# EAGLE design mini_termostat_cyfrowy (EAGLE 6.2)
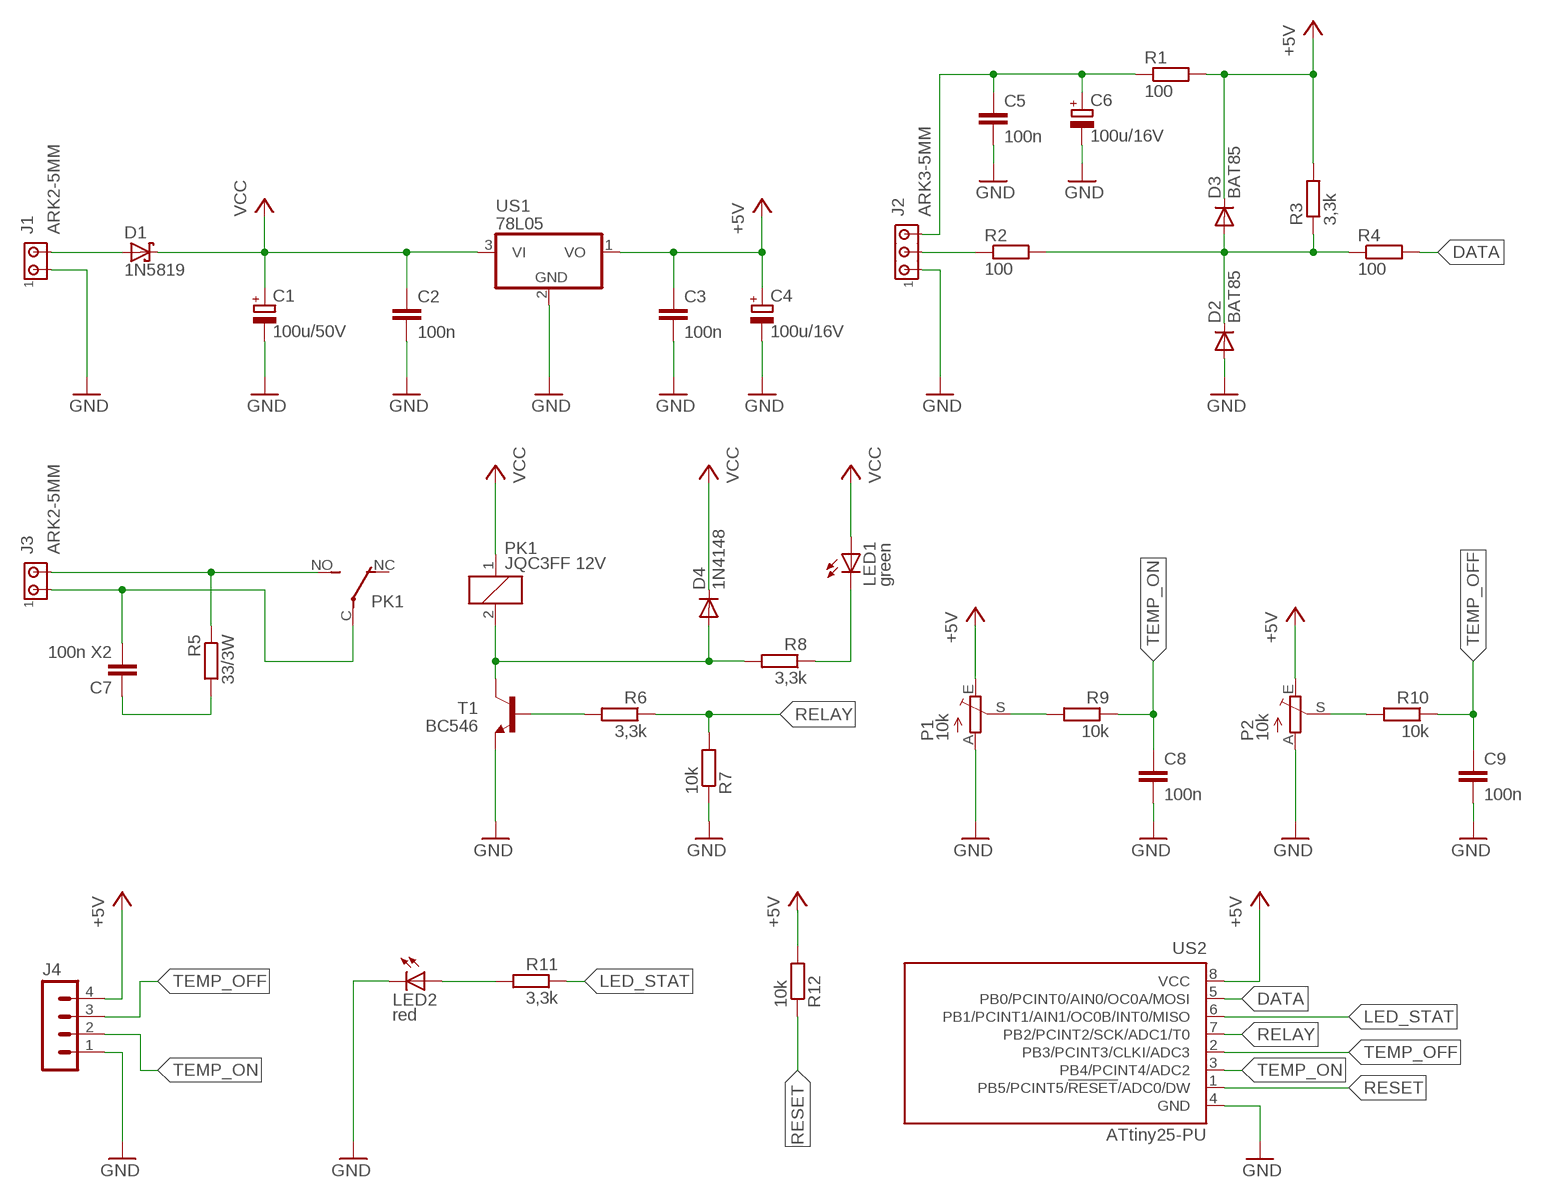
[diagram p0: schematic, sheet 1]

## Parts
C1  100u/50V  CPOL-EUE3.5-8  [E3,5-8]
C2  100n  C-EU050-025X075  [C050-025X075]
C3  100n  C-EU050-025X075  [C050-025X075]
C4  100u/16V  CPOL-EUE2.5-6  [E2,5-6]
C5  100n  C-EU050-025X075  [C050-025X075]
C6  100u/16V  CPOL-EUE2.5-5  [E2,5-5]
C7  100n X2  C-EU102_152-062X184  [C102_152-062X184]
C8  100n  C-EU050-025X075  [C050-025X075]
C9  100n  C-EU050-025X075  [C050-025X075]
D1  1N5819  1N5819-T  [DO41-7.6]
D2  BAT85  BAT81  [DO34-7]
D3  BAT85  BAT81  [DO34-7]
D4  1N4148  BAT81  [DO34-7]
J1  ARK2-5MM  [2PIN-5MM]
J2  ARK3-5MM  [3PIN-5MM]
J3  ARK2-5MM  [2PIN-5MM]
J4  MA04-1  [MA04-1]
LED1  green  LED5MM  [LED5MM]
LED2  red  LED5MM  [LED5MM]
P1  10k  TRIM_EU-B64Y  [B64Y]
P2  10k  TRIM_EU-B64Y  [B64Y]
PK1  JQC3FF 12V  PK_POJED-JQC-3FG  [PK_POJED_JQC-3FG]
R1  100  R-EU_0207/7  [0207/7]
R2  100  R-EU_0207/7  [0207/7]
R3  3,3k  R-EU_0204/2V  [0204V]
R4  100  R-EU_0207/7  [0207/7]
R5  33/3W  R-EU_0617/5V  [0617V]
R6  3,3k  R-EU_0207/7  [0207/7]
R7  10k  R-EU_0207/7  [0207/7]
R8  3,3k  R-EU_0204/2V  [0204V]
R9  10k  R-EU_0207/7  [0207/7]
R10  10k  R-EU_0207/7  [0207/7]
R11  3,3k  R-EU_0204/2V  [0204V]
R12  10k  R-EU_0204/2V  [0204V]
T1  BC546  BC546A  [TO92-EBC]
US1  78L05  7805L  [TO92]
US2  ATtiny25-PU  TINY13-20PU  [DIL08]

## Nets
+5V: C3.1 C4.+ D3.C J4.4 P1.E P2.E R1.2 R3.2 R12.2 US1.1(VO) US2.8(VCC)
DATA: R4.2 US2.5(PB0/PCINT0/AIN0/OC0A/MOSI)
GND: C1.- C2.2 C3.2 C4.- C5.2 C6.- C8.2 C9.2 D2.A J1.P$1 J2.P$1 J4.1 LED2.K(C) P1.A P2.A R7.1 T1.E US1.2(GND) US2.4(GND)
LED_STAT: R11.1 US2.6(PB1/PCINT1/AIN1/OC0B/INT0/MISO)
N$1: D1.A J1.P$2
N$2: J3.P$2 PK1.NO R5.1
N$3: P1.S R9.2
N$4: P2.S R10.2
N$5: LED1.K(C) R8.1
N$6: LED2.A R11.2
N$7: R6.2 T1.B
N$9: D4.A PK1.2 R8.2 T1.C
N$11: C7.2 J3.P$1 PK1.C(COM)
N$12: C7.1 R5.2
N$28: C5.1 C6.+ J2.P$3 R1.1
N$29: D2.C D3.A R2.2 R3.1 R4.1
N$30: J2.P$2 R2.1
RELAY: R6.1 R7.2 US2.7(PB2/PCINT2/SCK/ADC1/T0)
RESET: R12.1 US2.1(PB5/PCINT5/!RESET!/ADC0/DW)
TEMP_OFF: C9.1 J4.3 R10.1 US2.2(PB3/PCINT3/CLKI/ADC3)
TEMP_ON: C8.1 J4.2 R9.1 US2.3(PB4/PCINT4/ADC2)
VCC: C1.+ C2.1 D1.C D4.C LED1.A PK1.1 US1.3(VI)
Unconnected: PK1.NC

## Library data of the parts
C1 C4 C6 = rcl:CPOL-EU: POLARIZED CAPACITOR, European symbol
C2 C3 C5 C7-C9 = rcl:C-EU: CAPACITOR, European symbol
D1 = diode:1N581*: 1.0A SCHOTTKY BARRIER RECTIFIER
D2-D4 = diode:BAT81: DIODE
J1 J3 = zlacza_futrzak:ARK2: ARK 2
J2 = zlacza_futrzak:ARK3: ARK 3 Raster 5mm i 3,5mm
J4 = zlacza_futrzak:MA04-1: PIN HEADER; OC_FARNELL: unknown; OC_NEWARK: unknown
LED1 LED2 = led:LED: LED
P1 P2 = pot:TRIM_EU-: POTENTIOMETER
PK1 = inne_futrzak:PK_POJED
R1-R12 = rcl:R-EU_: RESISTOR, European symbol
T1 = transistor-npn:BC546*: NPN Transistor
US1 = linear:78*: Positive VOLTAGE REGULATOR Source: http://cache.national.com/ds/LM/LM78L05.pdf http://www.fairchildsemi.com/ds/LM/LM7805.pdf
US2 = atmel:TINY13: 8-bit AVR Microcontroller with 1K Bytes In-System Programmable Flash Source: http://www.atmel.com/dyn/resources/prod_documents/2535S.pdf; MPN: ATTINY13-20PU; OC_FARNELL: 9171550; OC_NEWARK: 96K6521

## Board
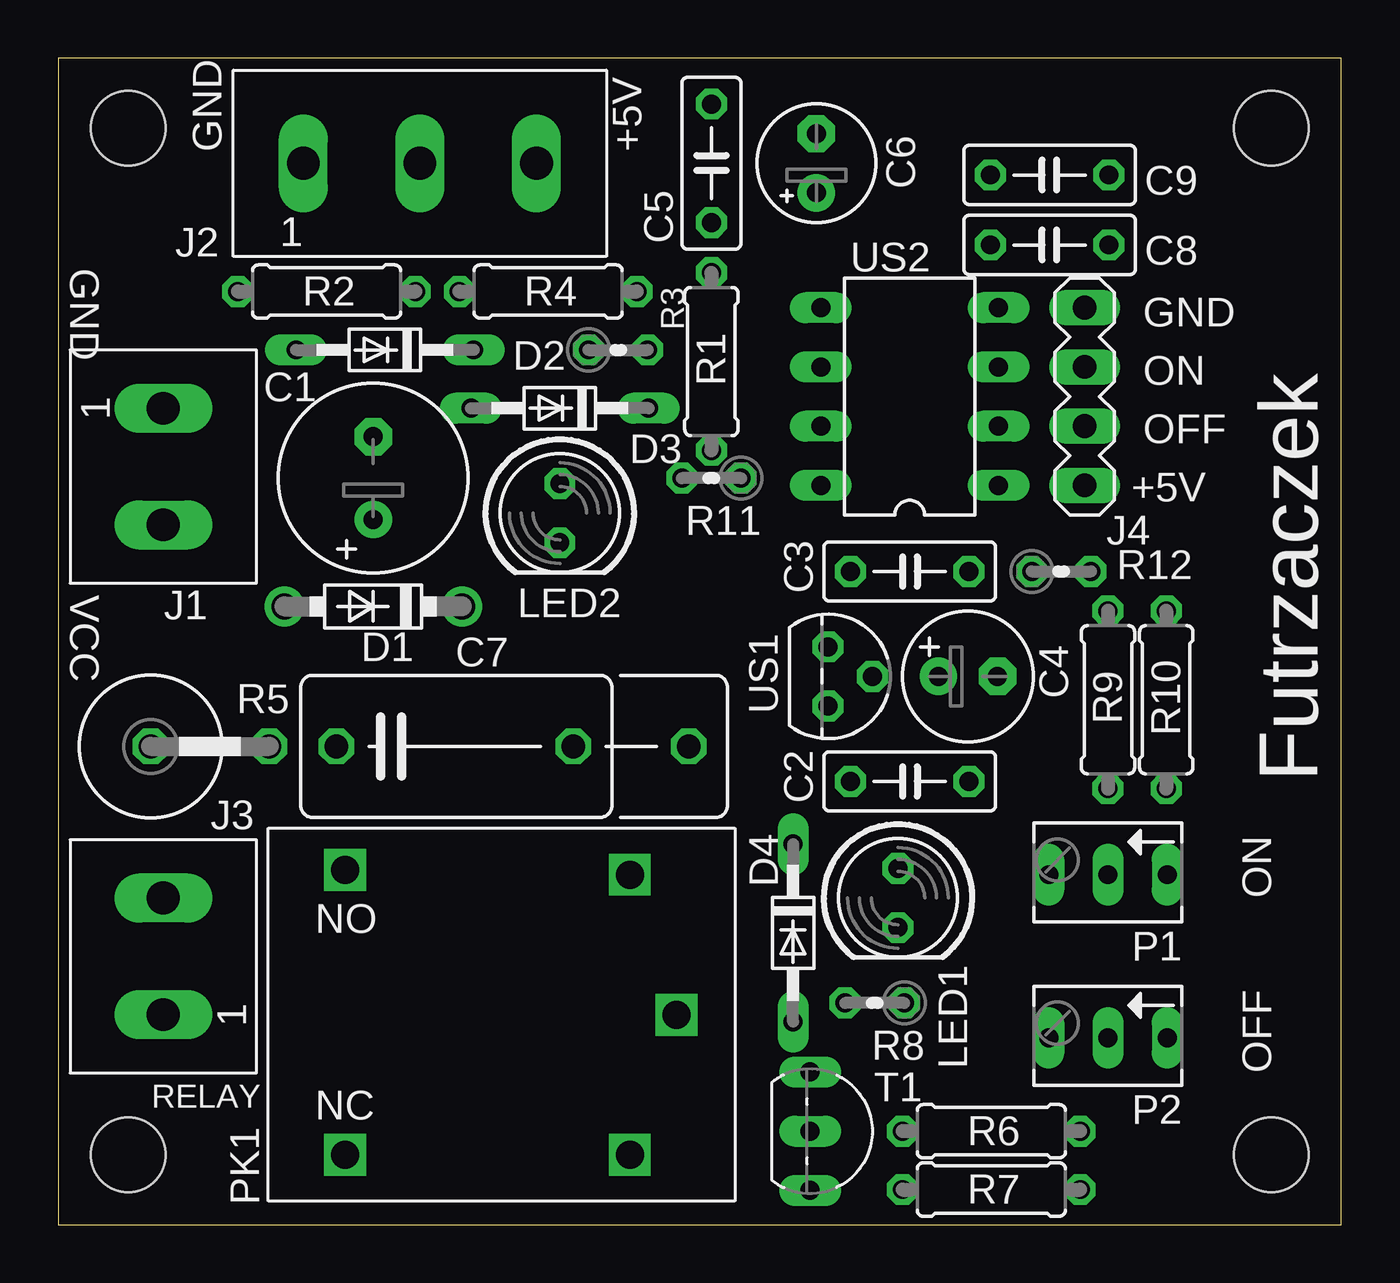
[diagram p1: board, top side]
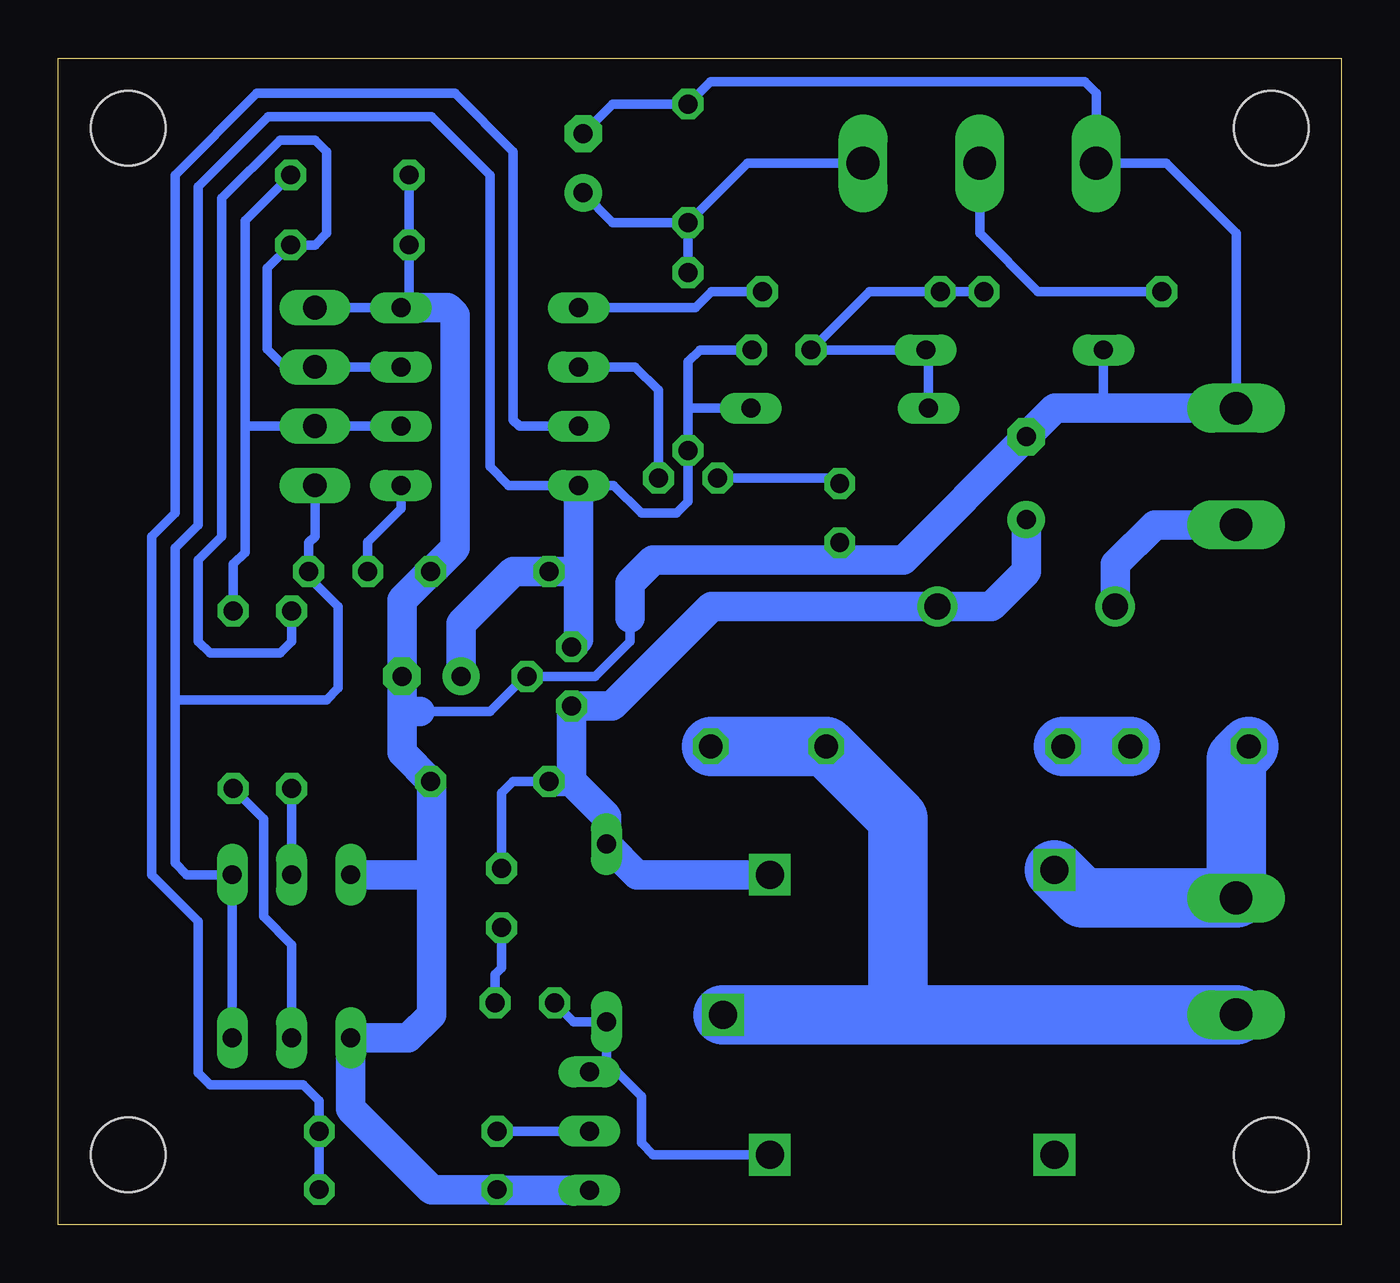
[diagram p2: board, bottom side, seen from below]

Size 55 x 50 mm. Coordinates in mm from the lower left corner, seen from the top.
Outline: 0,0 55,0 55,50 0,50 0,0
Copper layers (1*16): Top 0.035mm / dielectric 1.5mm / Bottom 0.035mm
Design rules: minimum track width 10mil, minimum drill 24mil, track to track 8mil, track to pad 8mil, pad to pad 8mil, via to via 8mil, smd to smd 8mil, copper to edge 20mil, drill to drill 8mil, minimum pad ring 10mil, minimum via ring 8mil, stop-mask expansion 4mil, vias tented up to drill 0mil, thermal gap 10mil
Holes 3.2 mm at 3,3 52,3 3,47 52,47

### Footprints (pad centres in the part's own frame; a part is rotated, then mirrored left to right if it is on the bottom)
E3,5-8 = drill 0.813 pad 1.6: + -1.778,0 | drill 0.813 pad 1.6 octagon: - 1.778,0
C050-025X075 = drill 0.813 octagon: 1 -2.54,0; 2 2.54,0
E2,5-6 = drill 0.813 pad 1.6: + -1.27,0 | drill 0.813 pad 1.6 octagon: - 1.27,0
E2,5-5 = drill 0.813 pad 1.6: + -1.27,0 | drill 0.813 pad 1.6 octagon: - 1.27,0
C102_152-062X184 = drill 1.016 octagon: 1 -5.08,0; 2 5.08,0; 3 10.033,0
DO41-7.6 = drill 1.1 pad 1.7: A 3.81,0; C -3.81,0
DO34-7 = drill 0.813 long: A 3.81,0; C -3.81,0
2PIN-5MM = drill 1.4 long: P$1 -2.5,0; P$2 2.5,0
3PIN-5MM = drill 1.4 long: P$1 -5,0; P$2 0,0; P$3 5,0
MA04-1 = drill 1.016 long: 1 -3.81,0; 2 -1.27,0; 3 1.27,0; 4 3.81,0
LED5MM = drill 0.813 octagon: A -1.27,0; K 1.27,0
B64Y = drill 0.813 long: A 2.54,0; E -2.54,0; S 0,0
PK_POJED_JQC-3FG = drill 1.2 square: 1 5.5,6; 2 5.5,-6; C 7.5,0; NC -6.7,-6; NO -6.7,6.2
0207/7 = drill 0.813 octagon: 1 -3.81,0; 2 3.81,0
0204V = drill 0.813 octagon: 1 -1.27,0; 2 1.27,0
0617V = drill 1.016 octagon: 1 -2.54,0; 2 2.54,0
TO92-EBC = drill 0.813 long: B 0,-1.27; C -2.54,-1.27; E 2.54,-1.27
TO92 = drill 0.813 octagon: 1 -1.27,0; 2 0,1.905; 3 1.27,0
DIL08 = drill 0.813 long: 1 -3.81,-3.81; 2 -1.27,-3.81; 3 1.27,-3.81; 4 3.81,-3.81; 5 3.81,3.81; 6 1.27,3.81; 7 -1.27,3.81; 8 -3.81,3.81

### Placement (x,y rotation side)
C1  13.5,32 90 top
C2  36.5,19 0 top
C3  36.5,28 0 top
C4  39,23.5 0 top
C5  28,45.5 90 top
C6  32.5,45.5 90 top
C7  17,20.5 0 top
C8  42.5,42 180 top
C9  42.5,45 180 top
D1  13.5,26.5 180 top
D2  14,37.5 180 top
D3  21.5,35 180 top
D4  31.5,12.5 270 top
J1  4.5,32.5 270 top
J2  15.5,45.5 0 top
J3  4.5,11.5 90 top
J4  44,35.5 270 top
LED1  36,14 270 top
LED2  21.5,30.5 270 top
P1  45,15 180 top
P2  45,8 180 top
PK1  19,9 0 top
R1  28,37 270 top
R2  11.5,40 0 top
R3  24,37.5 0 top
R4  21,40 0 top
R5  6.5,20.5 0 top
R6  40,4 180 top
R7  40,1.5 0 top
R8  35,9.5 180 top
R9  45,22.5 270 top
R10  47.5,22.5 270 top
R11  28,32 180 top
R12  43,28 0 top
T1  33.5,4 270 top
US1  33,23.5 270 top
US2  36.5,35.5 90 top

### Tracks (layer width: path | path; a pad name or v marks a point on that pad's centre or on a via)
+5V
  Bottom 0.406: J4.4 44,29.5 44.27,29.23 R12.2 44.27,27.77 43,26.5 43,23 43.5,22.5 50,22.5 | P2.E P1.E 49.5,15 50,15.5 50,22.5 | 50,22.5 50,29 49,30 49,44.5 46,47.5 39,47.5 36.5,45 36.5,32.5 35.69,31.69 US2.8 31.19,31.69 30,30.5 28.5,30.5 28,31 R1.2 28,35 | 28,35 28,37 27.5,37.5 R3.2 | D3.C 28,35
  Bottom 1.27: US2.8 32.69,28 | 32.69,28 32.69,25.08 US1.1 | 32.69,28 C3.1 35.5,28 37.73,25.77 C4.+
DATA
  Bottom 0.406: US2.5 27.69,39.31 27,40 R4.2
GND
  Bottom 0.406: 39.5,22 36.5,22 35,23.5 US1.2 32,23.5 30.5,25 30.5,26 | J4.1 US2.4 39.96,39.66 C8.2 C9.2 | LED2.K 21.5,28.5 | J1.P$1 4.5,42.5 7.5,45.5 J2.P$1 10.5,48.5 11,49 27.04,49 C5.2 31.23,48.04 C6.- | D2.A 10.19,35.19 10,35
  Bottom 1.27: 40.27,22 C4.- 40.27,26.77 C3.2 39,28 38,29 38,39 38.31,39.31 US2.4 | 40.27,22 40.27,20.23 C2.2 39,18.96 39,15 | 39.5,22 40.27,22 | J1.P$1 10,35 12.28,35 C1.- 18.78,28.5 21.5,28.5 29.5,28.5 30.5,27.5 30.5,26 | T1.E 36.15,1.46 R7.1 39,1.5 42.46,4.96 P2.A 40,8 39,9 39,15 | P1.A 39,15
LED_STAT
  Bottom 0.406: US2.6 30.27,36.77 29.27,35.77 R11.1
N$1
  Bottom 1.27: D1.A 9.69,28.31 8,30 J1.P$2
N$2
  Bottom 2.54: PK1.NO 11.1,14 J3.P$2 4.5,19.96 R5.1
N$3
  Bottom 0.406: P1.S R9.2
N$4
  Bottom 0.406: P2.S 45,12 46.2,13.2 46.2,17.39 R10.2
N$5
  Bottom 0.406: R8.1 36.27,10.73 36,11 LED1.K
N$6
  Bottom 0.406: R11.2 21.77,32 LED2.A
N$7
  Bottom 0.406: R6.2 T1.B
N$9
  Bottom 0.406: R8.2 32.92,8.69 D4.A 31.5,6.54 | T1.C 31.5,6.54 | 31.5,6.54 31.04,6.54 30,5.5 30,3.5 29.5,3 PK1.2
N$11
  Bottom 2.54: J3.P$1 19,9 | 19,9 PK1.C | 27,20.5 C7.2 19,17.42 19,9
N$12
  Bottom 2.54: R5.2 C7.1
N$28
  Bottom 0.406: R1.1 C5.1 | J2.P$3 25.46,45.5 C5.1 | C5.1 31.23,42.96 C6.+
N$29
  Bottom 0.406: R2.2 R4.1 20.23,40 R3.1 D2.C 17.69,37.38 D3.A
N$30
  Bottom 0.406: R2.1 13,40 15.5,42.5 J2.P$2
RELAY
  Bottom 0.406: US2.7 35.23,34.23 35.5,34.5 35.5,46 38,48.5 46.5,48.5 50,45 50,30.5 51,29.5 51,15 49,13 49,6.5 48.5,6 44.5,6 43.81,5.31 R6.1 R7.2
RESET
  Bottom 0.406: R12.1 41.73,29.27 40.31,30.69 US2.1
TEMP_OFF
  Bottom 0.406: US2.2 J4.3 47,34.23 | 47,34.23 47,28.81 47.5,28.31 R10.1 | 47,34.23 47,43.04 C9.1
TEMP_ON
  Bottom 0.406: US2.3 J4.2 45.27,36.77 46.04,37.54 46.04,41 C8.1 44,42 43.5,42.5 43.5,46 44,46.5 45.5,46.5 48,44 48,29.5 49,28.5 49,25 48.5,24.5 45.5,24.5 45,25 R9.1
VCC
  Bottom 0.406: LED1.A 36,18.5 35.5,19 C2.1
  Bottom 1.27: C1.+ 13.5,28 15,26.5 D1.C 27,26.5 31.27,22.23 US1.3 33,19 | PK1.1 30.19,15 D4.C 31.5,17.5 33,19 | 33,19 C2.1

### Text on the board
tPlace: GND | +5V | GND | GND | ON | OFF | +5V | VCC | Futrzaczek | ON | OFF | RELAY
